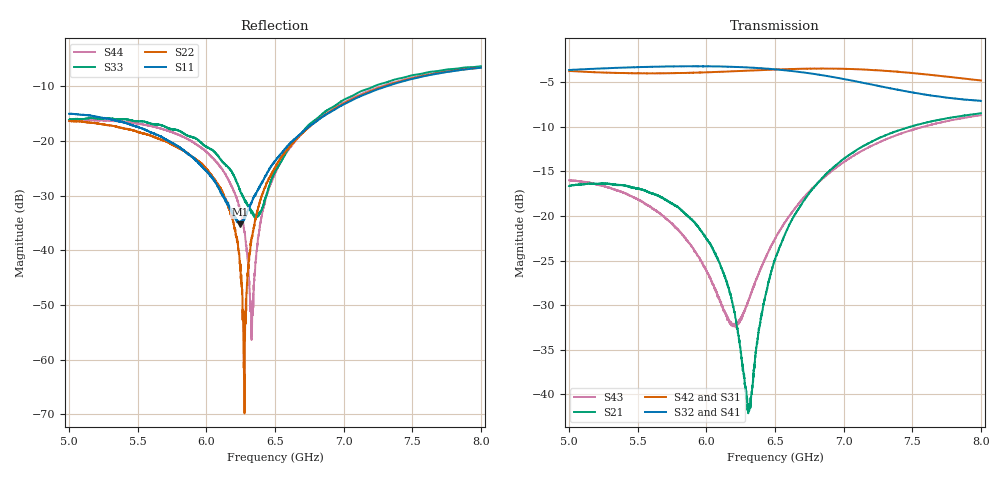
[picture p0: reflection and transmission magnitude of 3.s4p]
!Keysight Technologies,N5225A,MY51451420,A.10.40.12
!Date: Wednesday, May 11, 2016 11:07:50
!Correction: S11(Full 4 Port(1,2,3,4))
!S12(Full 4 Port(1,2,3,4))
!S13(Full 4 Port(1,2,3,4))
!S14(Full 4 Port(1,2,3,4))
!S21(Full 4 Port(1,2,3,4))
!S22(Full 4 Port(1,2,3,4))
!S23(Full 4 Port(1,2,3,4))
!S24(Full 4 Port(1,2,3,4))
!S31(Full 4 Port(1,2,3,4))
!S32(Full 4 Port(1,2,3,4))
!S33(Full 4 Port(1,2,3,4))
!S34(Full 4 Port(1,2,3,4))
!S41(Full 4 Port(1,2,3,4))
!S42(Full 4 Port(1,2,3,4))
!S43(Full 4 Port(1,2,3,4))
!S44(Full 4 Port(1,2,3,4))
!S4P File: Measurements: <S11,S12,S13,S14>,
!<S21,S22,S23,S24>,
!<S31,S32,S33,S34>,
!<S41,S42,S43,S44>:
# Hz S  dB  R 50
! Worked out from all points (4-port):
!   3201 points, 5 GHz to 8 GHz, reference 50 ohm
!   strongest paths, dB at 5 GHz, 5.75 GHz, 6.5 GHz, 7.25 GHz, 8 GHz:
!     S32: -3.6, -3.2, -3.5, -5.4, -7.1
!     S41: -3.6, -3.2, -3.5, -5.3, -7.1
!     S42: -3.7, -3.9, -3.6, -3.6, -4.8
!     S31: -3.8, -4.0, -3.6, -3.7, -4.8
!     S21: -16.6, -18.6, -24.8, -11.3, -8.5
!     S43: -16.0, -20.8, -22.5, -11.8, -8.7
!   lowest |S11| = -35.2 dB at 6.243 GHz (marker M1), VSWR 1.04, Z = 50.5 + j1.67 ohm
!   |S11| at or under -10 dB: start of sweep to 7.319 GHz; 7.319872 GHz to 7.320747 GHz (875.5 kHz wide, 0.012 % of centre)
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5e9  -15.05 11.7  -16.63 173.6  -3.78 10.3  -3.64 102.6
     -16.62 173.6  -16.40 -116.8  -3.60 -140.3  -3.71 129.0
     -3.77 10.3  -3.60 -140.3  -16.15 -130.6  -15.97 -78.9
     -3.65 102.5  -3.72 129.0  -15.98 -78.9  -16.34 -117.9
6.243125e9  -35.23 73.2  -34.67 25.1  -3.74 -164.7  -3.29 -74.0
            -34.45 25.3  -42.50 93.7  -3.28 72.4  -3.71 -16.4
            -3.73 -164.7  -3.28 72.4  -29.01 120.0  -31.87 -115.2
            -3.29 -74.0  -3.72 -16.5  -31.92 -114.7  -32.22 83.5
6.27875e9  -33.73 41.0  -38.69 39.3  -3.72 -169.8  -3.32 -79.2
           -38.91 40.1  -67.03 153.0  -3.30 68.1  -3.69 -20.8
           -3.72 -169.9  -3.30 68.1  -30.79 123.0  -30.60 -103.8
           -3.31 -79.2  -3.69 -20.8  -30.62 -103.5  -36.83 77.5
6.330312e9  -31.12 10.2  -39.73 110.5  -3.68 -177.4  -3.36 -86.7
            -39.73 111.6  -37.78 -91.0  -3.34 61.9  -3.66 -27.2
            -3.68 -177.4  -3.34 61.8  -32.95 148.6  -28.49 -94.6
            -3.36 -86.6  -3.65 -27.1  -28.46 -94.4  -52.89 -11.4
6.685625e9  -18.76 -90.4  -18.86 105.8  -3.49 129.7  -3.85 -137.7
            -18.86 105.7  -18.90 -134.9  -3.83 19.0  -3.47 -71.5
            -3.49 129.7  -3.83 19.0  -18.85 -152.1  -18.33 -109.4
            -3.84 -137.7  -3.46 -71.5  -18.32 -109.5  -18.99 -147.6
7.405625e9  -9.33 135.9  -10.36 -3.8  -3.89 19.9  -5.75 124.8
            -10.36 -3.8  -9.22 130.7  -5.85 -61.2  -3.81 -164.2
            -3.88 19.9  -5.85 -61.3  -8.61 128.3  -10.81 168.6
            -5.74 124.8  -3.81 -164.2  -10.81 168.7  -9.06 125.5
8e9  -6.67 40.0  -8.47 -87.0  -4.85 -67.8  -7.04 53.0
     -8.46 -87.0  -6.65 59.0  -7.07 -118.2  -4.77 121.9
     -4.85 -67.7  -7.07 -118.1  -6.37 58.6  -8.68 101.4
     -7.05 52.9  -4.78 121.9  -8.68 101.4  -6.49 58.7
